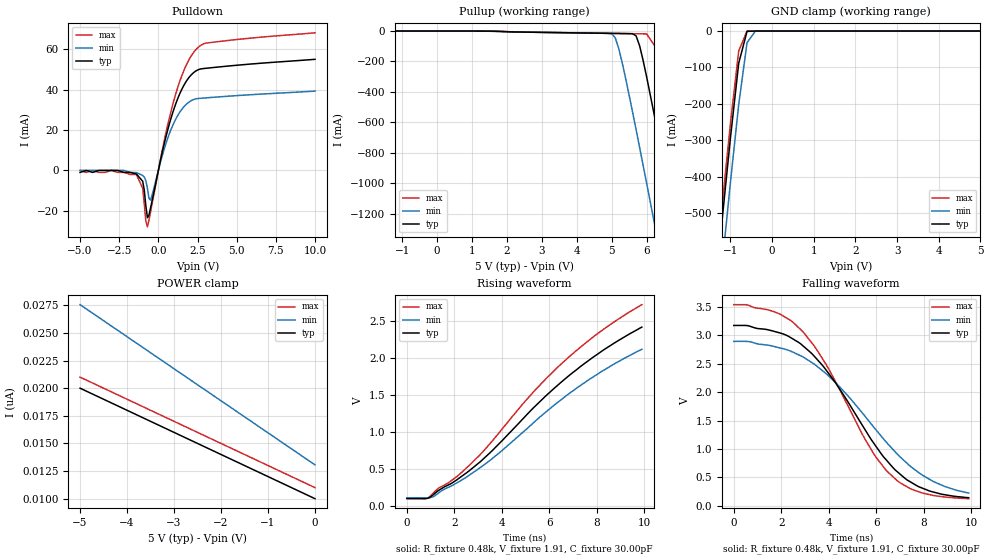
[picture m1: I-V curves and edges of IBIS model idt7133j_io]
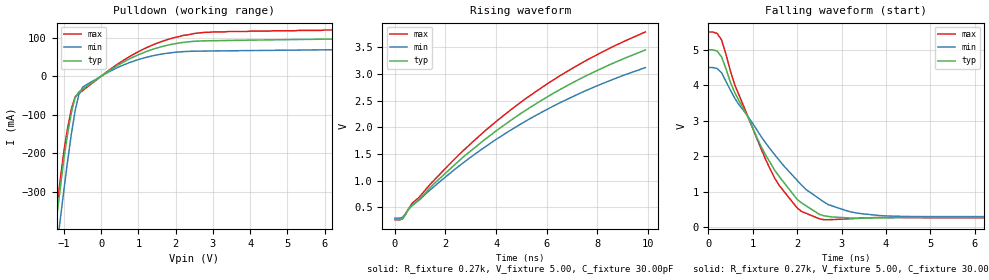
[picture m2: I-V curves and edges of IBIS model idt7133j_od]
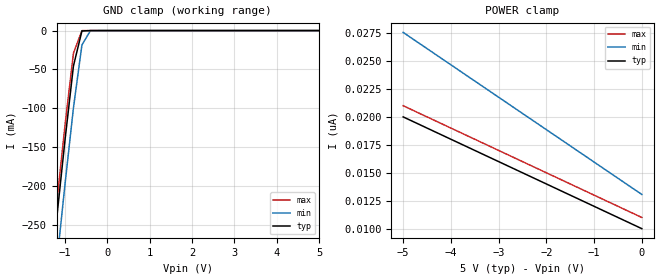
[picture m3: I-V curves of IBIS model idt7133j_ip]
| IBIS file idt7133j.ibs created by s2ibis2 version 1.1
| North Carolina State University Electronics Research Laboratory  1995
[IBIS ver]   2.1
[File name]   idt7133j.ibs
[File Rev]   1.0
[Date]   05/27/98
[Source]   Integrated Device Technology, Inc.
[Notes]   1.Temperatures: typ=25C, min=100C, max=0C 2.Cemos7 5vv
   process. 3.RRmp rates based on 50 ohm load.
[Disclaimer] Integrated Device Technology, Inc. ("IDT") hereby grants the
   user of this IBIS model a non-exclusive, nontransferable
   license to use this IBIS model under the following terms. The
   user is granted this license only to use the IBIS model and is
   not granted rights to sell, copy (except as needed to run the
   IBIS model), rent, lease or sub-license the IBIS model in
   whole or in part, or in modified form to anyone. The User may
   modify the IBIS model to suit its specific applications, but
   rights to derivative works and such modifications shall belong
   to IDT. This IBIS model is provided on an AS IS" basis and IDT
   makes absolutely no warranty with respect to the information
   contained herein. IDT DISCLAIMS AND CUSTOMER WAIVES ALL
   WARRANTIES, EXPRESS AND IMPLIED, INCLUDING WARRANTIES OF
   MERCHANTABILITY AND FITNESS FOR A PARTICULAR PURPOSE. THE
   ENTIRE RISK AS TO QUALITY AND PERFORMANCE IS WITH THE USER
   ACCORDINGLY, IN NO EVENT SHALL IDT BE LIABLE FOR ANY DIRECT OR
   INDIRECT DAMAGES, WHETHER IN CONTRACT OR TORT, INCLUDING ANY
   LOST PROFITS OR OTHER INCIDENTAL, CONSEQUENTIAL, EXEMPLARY, OR
   PUNITIVE DAMAGES ARISING OUT OF THE USE OR APPLICATION OF THE
   IBIS model. Further, IDT reserves the right to make changes
   without notice to any product herein to improve reliability,
   function, or design. IDT does not convey any license under
   patent rights or any other intellectual property rights,
   including those of third parties. IDT is not obligated to
   provide maintenance or support for the licensed IBIS model.
[Copyright]   Copyright 1998, Integrated Device Technology, Inc. all rights
   reserved
|   Component idt7133j
[Component]   idt7133j
[Manufacturer]   Integrated Device Technology
[Package]
| variable   typ   min   max
R_pkg   100.00m   50.00m   0.30
L_pkg   9.40nH   8.70nH   10.50nH
C_pkg   2.30pF   1.70pF   2.60pF
[Pin]  signal_name   model_name   R_pin   L_pin   C_pin
1   IO0L   idt7133j_io
2   IO1L   idt7133j_io
3   IO2L   idt7133j_io
4   IO3L   idt7133j_io
5   IO4L   idt7133j_io
6   IO5L   idt7133j_io
7   IO6L   idt7133j_io
8   IO7L   idt7133j_io
9   IO8L   idt7133j_io
10   IO9L   idt7133j_io
11   I10L   idt7133j_io
12   I11L   idt7133j_io
13   I12L   idt7133j_io
14   I13L   idt7133j_io
15   I14L   idt7133j_io
16   I15L   idt7133j_io
17   VDD   POWER
18   GND   GND
19   IO0R   idt7133j_io
20   IO1R   idt7133j_io
21   IO2R   idt7133j_io
22   IO3R   idt7133j_io
23   IO4R   idt7133j_io
24   IO5R   idt7133j_io
25   IO6R   idt7133j_io
26   IO7R   idt7133j_io
27   IO8R   idt7133j_io
28   IO9R   idt7133j_io
29   I10R   idt7133j_io
30   I11R   idt7133j_io
31   I12R   idt7133j_io
32   I13R   idt7133j_io
33   I14R   idt7133j_io
34   I15R   idt7133j_io
35   GND   GND
36   RWRUB   idt7133j_ip
37   RWRLB   idt7133j_ip
38   OER   idt7133j_ip
39   A10R   idt7133j_ip
40   A9R   idt7133j_ip
41   A8R   idt7133j_ip
42   A7R   idt7133j_ip
43   A6R   idt7133j_ip
44   A5R   idt7133j_ip
45   A4R   idt7133j_ip
46   A3R   idt7133j_ip
47   A2R   idt7133j_ip
48   A1R   idt7133j_ip
49   A0R   idt7133j_ip
50   BUSYR   idt7133j_od
51   CER   idt7133j_ip
52   CEL   idt7133j_ip
53   BUSYL   idt7133j_od
54   A0L   idt7133j_ip
55   A1L   idt7133j_ip
56   A2L   idt7133j_ip
57   A3L   idt7133j_ip
58   A4L   idt7133j_ip
59   A5L   idt7133j_ip
60   A6L   idt7133j_ip
61   A7L   idt7133j_ip
62   A8L   idt7133j_ip
63   A9L   idt7133j_ip
64   A10L   idt7133j_ip
65   OEL   idt7133j_ip
66   RWLLB   idt7133j_ip
67   RWLUB   idt7133j_ip
68   VDD   POWER
| Models and submodels in the file (3): idt7133j_io (I/O), idt7133j_od (Open_drain), idt7133j_ip (Input)
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| dsa  dsa   dummy_model
| oen  oen   dummy_model
| data data   dummy_model
|   Model idt7133j_io
[Model]   idt7133j_io
Model_type   I/O
Polarity   Inverting
Enable   Active-High
Vinl =  0.000V
Vinh =  5.000V
Vmeas =  1.500V
C_comp   3.00pF   NA   NA
[Temperature Range]   25.00   100.00   0.000
[Voltage Range]   5.00V   4.50V   5.50V
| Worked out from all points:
|   slope of the pulldown table from 0 to 0.75 V, typ, clamps not added: 30.8 ohm
|   slope of the pullup table from 0 to 0.75 V, typ, clamps not added: 14.3 kohm
|   GND clamp passes 1 mA (typ) near -0.60 V on its own axis
|   rising waveform, R_fixture 0.48k, V_fixture 1.91, C_fixture 30.00pF: 20-80 % time 4.64ns typ, 4.65ns min, 4.64ns max; typ from 0.101 V to 2.41 V
|   falling waveform, R_fixture 0.48k, V_fixture 1.91, C_fixture 30.00pF: 20-80 % time 3.02ns typ, 3.48ns min, 2.77ns max; typ from 3.17 V to 0.145 V
[Pulldown]
| voltage   I(typ)   I(min)   I(max)
-5V       -1mA       0A         0A
-1.4V     -1.8mA     -1.1mA     -2.1mA
-1V       -5.4mA     -2.5mA     -8.9mA
-800mV    -17.57mA   -5.1mA     -25.16mA
-700mV    -23.44mA   -8.9mA     -28mA
-500mV    -18.65mA   -14.74mA   -20.61mA
400mV     14.07mA    11.3mA     15.72mA
1V        30.62mA    23.72mA    35.01mA
1.7V      43.19mA    32.19mA    50.87mA
2.4V      49.36mA    35.51mA    59.96mA
3.1V      50.72mA    36.03mA    63.22mA
10V       55.11mA    39.34mA    68.26mA
[Pullup]
| voltage   I(typ)   I(min)   I(max)
-5V       0A         0A         0A
5V        -15.44mA   -18.12mA   -15.43mA
5.1V      -15.77mA   -43.15mA   -15.76mA
5.2V      -16.09mA   -113mA     -16.09mA
5.7V      -32.3mA    -649mA     -17.74mA
5.8V      -96.9mA    -765mA     -18.06mA
6V        -300mA     -999mA     -18.72mA
6.4V      -759mA     -1.472A    -155mA
6.8V      -1.233A    -1.951A    -602mA
7.2V      -1.712A    -2.431A    -1.074A
7.6V      -2.193A    -2.913A    -1.553A
10V       -5.103A    -5.822A    -4.458A
[GND_clamp]
| voltage   I(typ)   I(min)   I(max)
-5V       -5.098A    -5.211A    -5.062A
-1.4V     -754mA     -877mA     -714mA
-1.2V     -521mA     -645mA     -481mA
-1V       -295mA     -417mA     -255mA
-800mV    -88.43mA   -202mA     -54.69mA
-600mV    -965uA     -32.08mA   -205uA
-400mV    -431nA     -218uA     -26.4nA
5V        10nA       14.51nA    10nA
[POWER_clamp]
| voltage   I(typ)   I(min)   I(max)
-5V       20nA       27.56nA    21nA
-4.3V     18.6nA     25.53nA    19.6nA
-4.2V     18.4nA     25.24nA    19.4nA
0V        10nA       13.06nA    11nA
[Ramp]
| variable   typ   min   max
dV/dt_r   0.40/2.42n   0.35/2.62n   0.44/2.25n
dV/dt_f   1.35/4.21n   0.95/4.32n   1.68/4.15n
R_load = 50.00
[Rising Waveform]
R_fixture = 0.48k
V_fixture = 1.91
V_fixture_min = 1.72
V_fixture_max = 2.10
C_fixture = 30.00pF
R_dut = 100.00m
L_dut = 4.00nH
C_dut = 0.60pF
| time   V(typ)   V(min)   V(max)
0s        101mV      111mV      101mV
900ps     106mV      109mV      113mV
1.3ns     203mV      167mV      232mV
2.1ns     352mV      311mV      396mV
2.8ns     521mV      454mV      602mV
3.4ns     688mV      590mV      805mV
4.9ns     1.18V      998mV      1.383V
6.4ns     1.642V     1.409V     1.886V
8ns       2.041V     1.772V     2.317V
9.9ns     2.413V     2.114V     2.716V
[Falling Waveform]
R_fixture = 0.48k
V_fixture = 1.91
V_fixture_min = 1.72
V_fixture_max = 2.10
C_fixture = 30.00pF
R_dut = 100.00m
L_dut = 4.00nH
C_dut = 0.60pF
| time   V(typ)   V(min)   V(max)
0s        3.169V     2.889V     3.534V
1.8ns     3.054V     2.79V      3.394V
2.9ns     2.817V     2.621V     3.065V
3.5ns     2.579V     2.455V     2.742V
4.2ns     2.213V     2.2V       2.251V
5.9ns     1.102V     1.383V     914mV
6.9ns     598mV      906mV      440mV
7.7ns     359mV      616mV      263mV
8.4ns     246mV      432mV      186mV
9.9ns     145mV      227mV      128mV
|   Model idt7133j_od
[Model]   idt7133j_od
Model_type   Open_drain
Polarity   Inverting
Vinl =  0.000V
Vinh =  5.000V
Vmeas =  1.500V
C_comp   3.00pF   NA   NA
[Temperature Range]   25.00   100.00   0.000
[Voltage Range]   5.00V   4.50V   5.50V
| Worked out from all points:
|   slope of the pulldown table from 0 to 0.75 V, typ, clamps not added: 16.9 ohm
|   rising waveform, R_fixture 0.27k, V_fixture 5.00, C_fixture 30.00pF: 20-80 % time 5.47ns typ, 5.46ns min, 5.46ns max; typ from 0.268 V to 3.45 V
|   falling waveform, R_fixture 0.27k, V_fixture 5.00, C_fixture 30.00pF: 20-80 % time 1.22ns typ, 1.55ns min, 1.04ns max; typ from 5 V to 0.268 V
[Pulldown]
| voltage   I(typ)   I(min)   I(max)
-5V       -3.536A    -3.614A    -3.51A
-1.4V     -526mA     -610mA     -499mA
-1V       -214mA     -294mA     -193mA
-900mV    -148mA     -219mA     -134mA
-800mV    -94.13mA   -149mA     -84.27mA
-700mV    -55.21mA   -89.71mA   -54.19mA
-600mV    -40.85mA   -47.89mA   -44.87mA
-500mV    -33.95mA   -29.1mA    -37.5mA
600mV     36.75mA    29.16mA    41.36mA
1.6V      76.1mA     57.03mA    89.24mA
3V        92.17mA    65.46mA    115mA
10V       100mA      71.62mA    124mA
[Ramp]
| variable   typ   min   max
dV/dt_r   2.14/0.16n   1.72/0.17n   2.46/0.16n
dV/dt_f   2.14/0.16n   1.72/0.19n   2.46/0.15n
R_load = 50.00
[Rising Waveform]
R_fixture = 0.27k
V_fixture = 5.00
V_fixture_min = 4.50
V_fixture_max = 5.50
C_fixture = 30.00pF
R_dut = 100.00m
L_dut = 4.00nH
C_dut = 0.60pF
| time   V(typ)   V(min)   V(max)
0s        268mV      296mV      267mV
300ps     284mV      310mV      283mV
700ps     541mV      538mV      585mV
900ps     623mV      610mV      660mV
2.6ns     1.398V     1.295V     1.515V
3.7ns     1.822V     1.674V     1.987V
5.1ns     2.295V     2.094V     2.512V
6.1ns     2.59V      2.355V     2.837V
7.6ns     2.973V     2.696V     3.262V
9.9ns     3.447V     3.117V     3.785V
[Falling Waveform]
R_fixture = 0.27k
V_fixture = 5.00
V_fixture_min = 4.50
V_fixture_max = 5.50
C_fixture = 30.00pF
R_dut = 100.00m
L_dut = 4.00nH
C_dut = 0.60pF
| time   V(typ)   V(min)   V(max)
0s        5V         4.5V       5.5V
200ps     4.962V     4.471V     5.462V
300ps     4.801V     4.354V     5.278V
600ps     3.784V     3.627V     4.002V
1.2ns     2.25V      2.536V     2.177V
1.5ns     1.596V     2.036V     1.373V
2.1ns     684mV      1.185V     442mV
2.7ns     301mV      636mV      210mV
3.9ns     263mV      322mV      272mV
9.9ns     268mV      296mV      267mV
|   Model idt7133j_ip
[Model]   idt7133j_ip
Model_type   Input
Vinl =  0.800V
Vinh =  2.200V
Vmeas =  1.500V
C_comp   3.00pF   NA   NA
[Temperature Range]   25.00   100.00   0.000
[Voltage Range]   5.00V   4.50V   5.50V
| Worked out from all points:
|   GND clamp passes 1 mA (typ) near -0.60 V on its own axis
[GND_clamp]
| voltage   I(typ)   I(min)   I(max)
-5V       -2.333A    -2.387A    -2.316A
-1.4V     -351mA     -409mA     -332mA
-1.2V     -244mA     -302mA     -225mA
-1V       -141mA     -198mA     -122mA
-800mV    -45.44mA   -99.28mA   -29.09mA
-600mV    -508uA     -18.46mA   -96.66uA
-400mV    -430nA     -140uA     -26.4nA
5V        10nA       14.51nA    10nA
[POWER_clamp]
| voltage   I(typ)   I(min)   I(max)
-5V       20nA       27.56nA    21nA
-4.3V     18.6nA     25.53nA    19.6nA
-4.2V     18.4nA     25.24nA    19.4nA
0V        10nA       13.06nA    11nA
